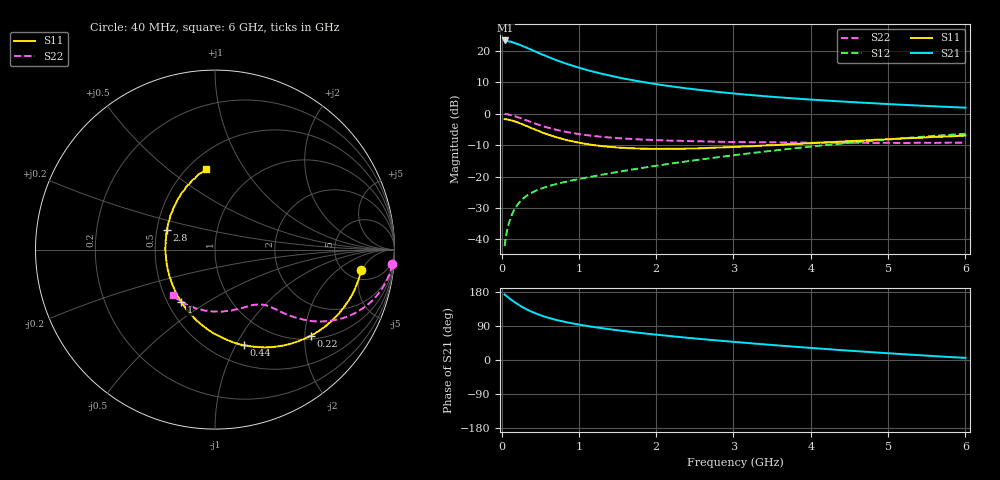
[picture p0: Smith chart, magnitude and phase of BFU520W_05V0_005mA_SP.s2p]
! Filename:  P:\Prog\Test\Noise\ATS_data\Testdata_Net\Run2\BFU520W_APM2013_06_A05_05p0V_005mA_SP_CM01_D.s2p
! Date/Time: Tue 26/Mar/2013 18:01:40
! BFU520W_APM2013_06_A05_05p0V_1to20mA_SP_CM01_Bias4_R.s2p
! MDIF S-parameter v. bias file
! BFU520W_APM2013_06_A05_05p0V_1to20mA_SP_CM01
! Date/time Thu Mar 21 14:22:37 2013
! VAR V_out= 5.0010
! VAR I_out= 4.9950
! VAR V_in= 0.8288
! VAR I_in= 0.0560
! Device data file deembeded for feedlines and parallel
! Original file: \Run2\BFU520W_APM2013_06_A05_05p0V_005mA_SP_CM01_R.s2p
! Feed-files: PR019V01_070313_Feed1.s2p, PR019V01_070313_Feed2.s2p
! Parallel-file: PR019V01_070313_Par.s2p
# MHz S MA R 50
!  Freq-MHz  S11-mag  S11-arg  S21-mag  S21-arg  S12-mag  S12-arg  S22-mag  S22-arg
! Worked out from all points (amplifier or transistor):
!   98 points, 40 MHz to 6 GHz, reference 50 ohm
!   highest |S21| = 23.4 dB at 50 MHz (marker M1)
!   |S21| within 3 dB of that: start of sweep to 388.1 MHz
!   unconditionally stable (mu >= 1): 1.813 GHz to 3.007 GHz
!   at 300 MHz: K = 0.33, MSG = 24.0 dB, |S12| = -26.6 dB
!   at 1.6 GHz: K = 0.97, MSG = 14.6 dB, |S12| = -18.1 dB
!   at 6 GHz: K = 0.86, MSG = 4.2 dB, |S12| = -6.4 dB
!   S11 on the Smith chart (normalised r, x): 40 MHz: 6.75, -4.80; 220 MHz: 1.09, -2.15; 440 MHz: 0.70, -1.08; 1 GHz: 0.59, -0.39; 2.8 GHz: 0.57, +0.13; 6 GHz: 0.61, +0.68
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40  0.8218 -8.1  14.73 172.9  0.007758 84.9  0.9909 -4.7
50  0.8197 -10.1  14.74 171.2  0.009587 84.6  0.9884 -5.9
90  0.8046 -18.0  14.26 164.6  0.01699 80.3  0.971 -10.5
140  0.7757 -27.6  13.82 156.9  0.0255 75.6  0.9386 -15.7
220  0.7189 -41.8  12.79 145.9  0.03725 69.3  0.873 -22.8
260  0.688 -48.2  12.2 140.9  0.04228 66.7  0.8386 -25.9
320  0.6402 -57.5  11.39 134.2  0.04877 63.5  0.7866 -29.7
380  0.5963 -65.7  10.54 128.3  0.05429 61.1  0.7381 -32.8
440  0.5558 -73.3  9.792 123.1  0.05919 59.3  0.6955 -35.1
550  0.4902 -85.7  8.573 114.9  0.0665 57.3  0.6268 -38.5
700  0.4261 -100.0  7.232 106.2  0.07531 56.1  0.5591 -41.3
850  0.3794 -112.3  6.213 99.3  0.08331 56.0  0.5102 -43.1
1000  0.3464 -123.1  5.436 93.5  0.09105 56.5  0.4746 -44.4
1050  0.338 -126.4  5.214 91.7  0.09362 56.8  0.4651 -44.9
1250  0.31 -138.9  4.485 85.4  0.1043 57.7  0.435 -46.5
1450  0.2943 -149.8  3.94 79.8  0.1153 58.6  0.4137 -48.2
2050  0.2759 -176.7  2.902 65.8  0.1514 60.4  0.3786 -54.3
2800  0.2895 158.1  2.227 51.5  0.2028 60.1  0.3582 -65.1
3100  0.2997 149.9  2.051 46.2  0.2257 59.4  0.3546 -69.8
4100  0.3459 127.8  1.656 30.4  0.3087 54.6  0.3443 -88.8
5200  0.4054 108.6  1.389 15.2  0.4081 46.2  0.3416 -113.3
6000  0.45 96.7  1.25 5.6  0.4799 38.7  0.3449 -133.2
